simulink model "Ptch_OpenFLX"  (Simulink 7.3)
settings: Solver=ode45  StartTime=0.0  StopTime=300  RelTol=1e-3
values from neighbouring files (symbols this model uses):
  Aac = [    [actuator.m]
  Bac = [    [actuator.m]
  Cac = [    [actuator.m]
  Cza = -0.343    [init.m]
  d2r = pi/180    (= 0.0174532925199)    [init.m]    (also in run.m; LQR_Des.m)
  Dac = [    [actuator.m]
  Kc = [12.6, 3.15, -0.3, 0.37]*0.127    [init.m]
  Mass = 9580    [init.m]
  Qbar = 228    [init.m]
  Sref = 47.3    [init.m]
  Thr = 363305    [init.m]
undefined symbols (not defined in the file or in its folder): Avf, Bvf, Cvf, Dvf

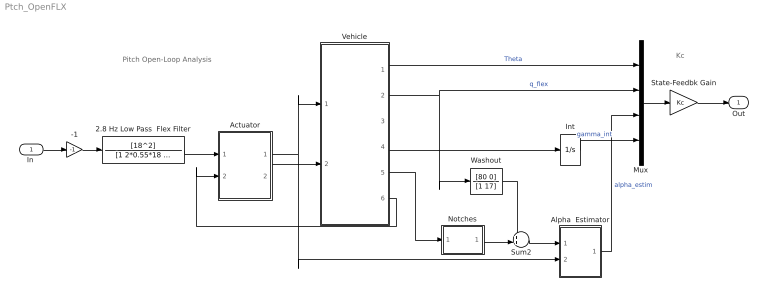
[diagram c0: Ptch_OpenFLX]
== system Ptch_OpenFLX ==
  note: Pitch Open-Loop Analysis
  note: Kc
  "In " : Inport  OutDataType=sfix(16)  OutScaling=2^0
  -1 : Gain  Gain=-1  ParameterDataType=sfix(16)  ParameterScaling=2^0  OutDataType=sfix(16)  OutScaling=2^0
  2.8 Hz Low Pass  Flex Filter : TransferFcn  Numerator=[18^2]  Denominator="[1 2*0.55*18  18^2]"
  Actuator : Subsystem
  Alpha  Estimator : Subsystem
  Int : Integrator
  Mux : Mux
  Notches : Subsystem
  State-Feedbk Gain : Gain  Gain=Kc  Multiplication=Matrix(K*u)  ParameterDataType=sfix(16)  ParameterScaling=2^0  OutDataType=sfix(16)  OutScaling=2^0
  Sum2 : Sum  Inputs=++|  OutDataType=sfix(16)  OutScaling=2^0
  Vehicle : Subsystem
  Washout : TransferFcn  Numerator=[80 0]  Denominator=[1 17]
  Out : Outport  OutDataType=sfix(16)  OutScaling=2^0
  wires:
  Actuator/1(Dy) -> Vehicle/1(Dy), Alpha  Estimator/2(delta)
  Int/1 -> Mux/4  "gamma_int"
  Mux/1 -> State-Feedbk Gain/1
  Sum2/1 -> Alpha  Estimator/1(Zdd)
  Alpha  Estimator/1(alphat) -> Mux/3  "alpha_estim"
  Vehicle/1(theta) -> Mux/1  "Theta"
  Vehicle/5(Zdd-flex) -> Notches/1(In)
  Vehicle/4(gama) -> Int/1
  Vehicle/2(q-flex) -> Mux/2, Washout/1  "q_flex"
  Washout/1 -> Sum2/1
  -1/1 -> 2.8 Hz Low Pass  Flex Filter/1
  Notches/1(Ou) -> Sum2/2
  2.8 Hz Low Pass  Flex Filter/1 -> Actuator/1(Dyc)
  State-Feedbk Gain/1 -> Out/1
  "In "/1 -> -1/1
  Actuator/2(Dy_dd) -> Vehicle/2(Dy_dd)
  Vehicle/6(TLy) -> Actuator/2(TLy)

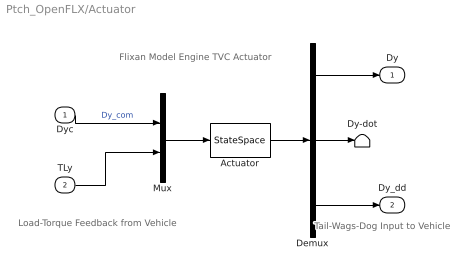
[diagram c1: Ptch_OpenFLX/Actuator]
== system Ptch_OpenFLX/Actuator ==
  note: Flixan Model Engine TVC Actuator
  note: Load-Torque Feedback from Vehicle
  note: Tail-Wags-Dog Input to Vehicle
  Dyc : Inport  OutDataType=sfix(16)  OutScaling=2^0
  TLy : Inport  Port=2  OutDataType=sfix(16)  OutScaling=2^0
  Actuator : StateSpace  A=Aac  B=Bac  C=Cac  D=Dac
  Demux : Demux  Outputs=3
  Dy-dot : Terminator
  Mux : Mux  Inputs=2
  Dy : Outport  OutDataType=sfix(16)  OutScaling=2^0
  Dy_dd : Outport  Port=2  OutDataType=sfix(16)  OutScaling=2^0
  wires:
  TLy/1 -> Mux/2
  Demux/3 -> Dy_dd/1
  Demux/1 -> Dy/1
  Dyc/1 -> Mux/1  "Dy_com"
  Demux/2 -> Dy-dot/1
  Actuator/1 -> Demux/1
  Mux/1 -> Actuator/1

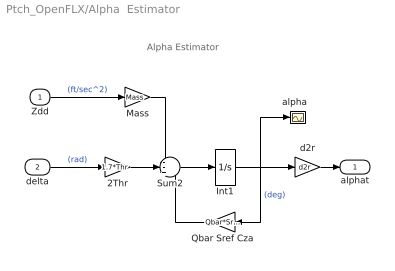
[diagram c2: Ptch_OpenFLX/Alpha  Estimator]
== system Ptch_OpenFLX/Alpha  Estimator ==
  note: Alpha Estimator
  Zdd : Inport  OutDataType=sfix(16)  OutScaling=2^0
  delta : Inport  Port=2  OutDataType=sfix(16)  OutScaling=2^0
  2Thr : Gain  Gain=1.7*Thr  ParameterDataType=sfix(16)  ParameterScaling=2^0  OutDataType=sfix(16)  OutScaling=2^0
  Int1 : Integrator
  Mass : Gain  Gain=Mass  ParameterDataType=sfix(16)  ParameterScaling=2^0  OutDataType=sfix(16)  OutScaling=2^0
  Qbar Sref Cza : Gain  Gain=Qbar*Sref*Cza  ParameterDataType=sfix(16)  ParameterScaling=2^0  OutDataType=sfix(16)  OutScaling=2^0
  Sum2 : Sum  Inputs=--+  OutDataType=sfix(16)  OutScaling=2^0
  "alpha  " : Scope
  d2r : Gain  Gain=d2r  ParameterDataType=sfix(16)  ParameterScaling=2^0  OutDataType=sfix(16)  OutScaling=2^0
  alphat : Outport  OutDataType=sfix(16)  OutScaling=2^0
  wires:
  d2r/1 -> alphat/1
  Mass/1 -> Sum2/1
  Zdd/1 -> Mass/1  "(ft/sec^2)"
  delta/1 -> 2Thr/1  "(rad)"
  Qbar Sref Cza/1 -> Sum2/3
  Int1/1 -> "alpha  "/1, d2r/1, Qbar Sref Cza/1  "(deg)"
  2Thr/1 -> Sum2/2
  Sum2/1 -> Int1/1

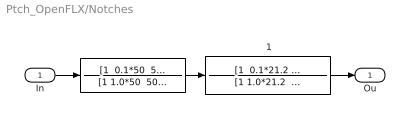
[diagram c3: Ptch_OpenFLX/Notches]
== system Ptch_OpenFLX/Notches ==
  In : Inport
  " " : TransferFcn  Numerator="[1  0.1*50  50^2]"  Denominator="[1 1.0*50  50^2]"
  " 1" : TransferFcn  Numerator="[1  0.1*21.2  21.2^2]"  Denominator="[1 1.0*21.2  21.2^2]"
  Ou : Outport
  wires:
  " "/1 -> " 1"/1
  In/1 -> " "/1
  " 1"/1 -> Ou/1

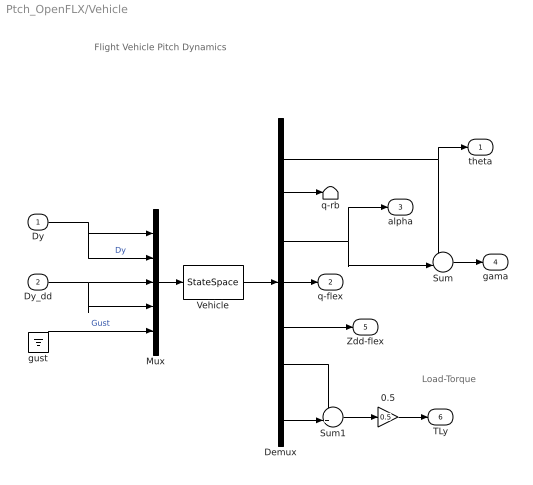
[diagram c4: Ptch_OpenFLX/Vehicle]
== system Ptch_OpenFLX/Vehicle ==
  note: Load-Torque
  note: Flight Vehicle Pitch Dynamics
  Dy : Inport  OutDataType=sfix(16)  OutScaling=2^0
  Dy_dd : Inport  Port=2  OutDataType=sfix(16)  OutScaling=2^0
  0.5 : Gain  Gain=0.5  ParameterDataType=sfix(16)  ParameterScaling=2^0  OutDataType=sfix(16)  OutScaling=2^0
  Demux : Demux  Outputs=7
  Mux : Mux  Inputs=5
  Sum : Sum  Inputs=+-|  OutDataType=sfix(16)  OutScaling=2^0
  Sum1 : Sum  Inputs=++|  OutDataType=sfix(16)  OutScaling=2^0
  Vehicle : StateSpace  A=Avf  B=Bvf  C=Cvf  D=Dvf
  gust : Ground
  q-rb : Terminator
  theta : Outport  OutDataType=sfix(16)  OutScaling=2^0
  q-flex : Outport  Port=2  OutDataType=sfix(16)  OutScaling=2^0
  alpha : Outport  Port=3  OutDataType=sfix(16)  OutScaling=2^0
  gama : Outport  Port=4  OutDataType=sfix(16)  OutScaling=2^0
  Zdd-flex : Outport  Port=5  OutDataType=sfix(16)  OutScaling=2^0
  TLy : Outport  Port=6  OutDataType=sfix(16)  OutScaling=2^0
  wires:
  0.5/1 -> TLy/1
  Sum1/1 -> 0.5/1
  Demux/2 -> q-rb/1
  Demux/4 -> q-flex/1
  Sum/1 -> gama/1
  Demux/6 -> Sum1/1
  Demux/7 -> Sum1/2
  Demux/5 -> Zdd-flex/1
  Demux/3 -> Sum/2, alpha/1
  Demux/1 -> Sum/1, theta/1
  Dy_dd/1 -> Mux/4, Mux/3
  gust/1 -> Mux/5  "Gust"
  Dy/1 -> Mux/2, Mux/1  "Dy"
  Vehicle/1 -> Demux/1
  Mux/1 -> Vehicle/1
